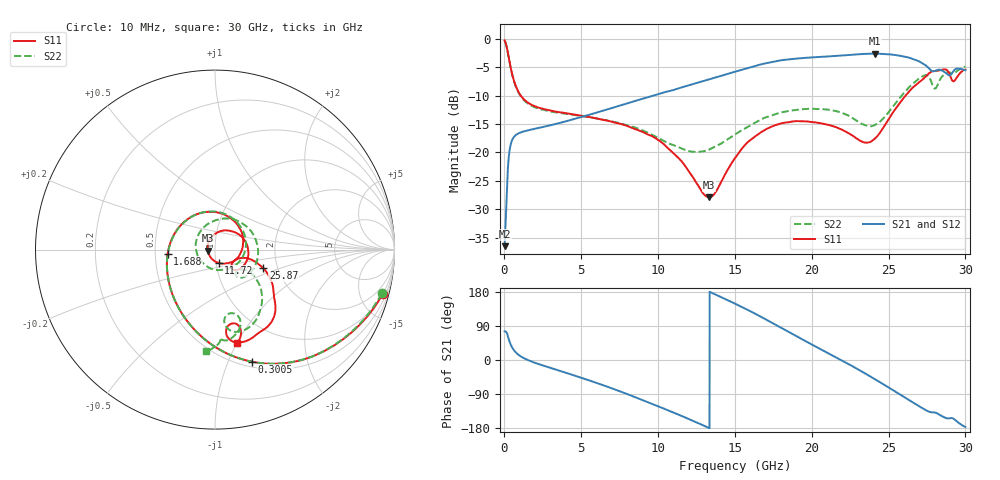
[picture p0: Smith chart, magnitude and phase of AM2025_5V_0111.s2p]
!Keysight Technologies,N5245B,MY58422270,A.16.20.02
!Date: Tuesday, July 14, 2026 01:05:45
!Correction: S11(C  2-Port  )
!S21(C  2-Port  )
!S12(C  2-Port  )
!S22(C  2-Port  )
!S2P File: Measurements: S11, S21, S12, S22:
# Hz S  dB  R 50
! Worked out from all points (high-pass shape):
!   3201 points, 10 MHz to 30 GHz, reference 50 ohm
!   highest |S21| = -2.62 dB at 24.13 GHz (marker M1); lowest = -36.5 dB at 10 MHz (marker M2)
!   |S21| within 3 dB of the highest: 15.24 GHz to 27.79 GHz (12.55 GHz wide, 58.3 % of centre); 29.24 GHz to end of sweep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
!   lowest |S11| = -27.9 dB at 13.34 GHz (marker M3), VSWR 1.08, Z = 46.2 - j0.509 ohm
!   |S11| at or under -10 dB: 1.062 GHz to 26.11 GHz (25.05 GHz wide, 184 % of centre)
!   |S22| runs from -19.9 to -0.4 dB; largest |S21 - S12| = 0.0087
!   S11 on the Smith chart (normalised r, x): 10 MHz: 1.03, -7.57; 300.5 MHz: 0.56, -1.23; 1.688 GHz: 0.58, -0.03; 11.72 GHz: 1.03, -0.15; 25.87 GHz: 1.68, -0.38; 30 GHz: 0.68, -1.00
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1e7  -0.30 -14.8  -36.48 75.8  -36.16 42.8  -0.36 -14.8
3.005281e8  -3.62 -71.6  -20.31 52.2  -20.28 52.2  -3.67 -72.1
4.785938e8  -5.98 -96.7  -17.97 34.7  -17.98 34.8  -6.04 -97.4
7.128906e8  -8.15 -119.7  -17.00 21.2  -16.98 21.2  -8.23 -120.8
1.687566e9  -11.51 -174.4  -16.01 -2.9  -16.01 -2.8  -11.67 -177.7
3.243297e9  -12.77 136.3  -15.05 -24.1  -15.05 -24.1  -12.90 129.6
5.014581e9  -13.54 92.6  -13.76 -47.0  -13.76 -47.1  -13.59 82.7
7.563731e9  -14.97 34.4  -11.71 -83.4  -11.71 -83.4  -14.89 19.0
1.000979e10  -17.80 -24.8  -9.75 -122.1  -9.75 -122.1  -17.43 -48.9
1.172484e10  -22.23 -75.0  -8.40 -151.0  -8.40 -151.1  -19.51 -109.0
1.333681e10  -27.89 -172.2  -7.13 -179.8  -7.13 -179.8  -19.47 178.5
1.5005e10  -20.99 87.9  -5.80 148.7  -5.80 148.7  -16.84 111.0
1.77697e10  -15.07 13.3  -3.91 90.3  -3.91 90.3  -13.12 33.3
2.000958e10  -14.65 -24.9  -3.28 40.7  -3.28 40.7  -12.32 -11.6
2.221197e10  -16.33 -47.4  -2.92 -6.7  -2.92 -6.8  -13.28 -46.0
2.413321e10  -17.48 -23.6  -2.62 -51.1  -2.62 -51.2  -15.15 -40.3
2.500479e10  -14.17 -14.9  -2.72 -72.5  -2.72 -72.6  -12.90 -32.9
2.5867e10  -10.79 -21.2  -3.05 -93.8  -3.05 -93.9  -9.96 -38.6
2.726341e10  -7.07 -41.2  -4.41 -128.6  -4.40 -128.8  -6.53 -65.7
2.803191e10  -5.65 -59.0  -5.66 -138.7  -5.66 -138.8  -8.76 -76.4
2.899721e10  -6.46 -82.4  -6.42 -153.3  -6.40 -153.5  -5.94 -85.3
3e10  -5.44 -77.0  -5.53 -176.6  -5.52 -176.7  -4.89 -94.9
